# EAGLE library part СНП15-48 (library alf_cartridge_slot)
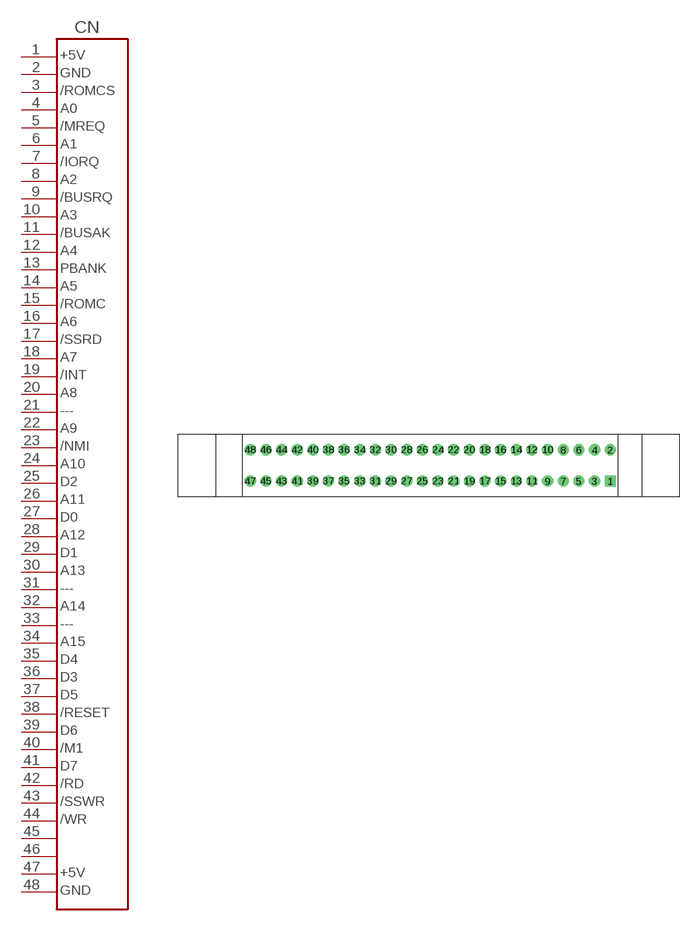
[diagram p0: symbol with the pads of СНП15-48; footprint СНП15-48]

Designator prefix CN

## СНП15-48  [СНП15-48]
1  1
2  2
3  3
4  4
5  5
6  6
7  7
8  8
9  9
10  10
11  11
12  12
13  13
14  14
15  15
16  16
17  17
18  18
19  19
20  20
21  21
22  22
23  23
24  24
25  25
26  26
27  27
28  28
29  29
30  30
31  31
32  32
33  33
34  34
35  35
36  36
37  37
38  38
39  39
40  40
41  41
42  42
43  43
44  44
45  45
46  46
47  47
48  48

## Footprint СНП15-48 (pad centres in mm)
drill 1 pad 1.778 square: 1 29,-2.5
drill 1 pad 1.778: 2 29,2.5; 3 26.5,-2.5; 4 26.5,2.5; 5 24,-2.5; 6 24,2.5; 7 21.5,-2.5; 8 21.5,2.5; 9 19,-2.5; 10 19,2.5; 11 16.5,-2.5; 12 16.5,2.5; 13 14,-2.5; 14 14,2.5; 15 11.5,-2.5; 16 11.5,2.5; 17 9,-2.5; 18 9,2.5; 19 6.5,-2.5; 20 6.5,2.5; 21 4,-2.5; 22 4,2.5; 23 1.5,-2.5; 24 1.5,2.5; 25 -1,-2.5; 26 -1,2.5; 27 -3.5,-2.5; 28 -3.5,2.5; 29 -6,-2.5; 30 -6,2.5; 31 -8.5,-2.5; 32 -8.5,2.5; 33 -11,-2.5; 34 -11,2.5; 35 -13.5,-2.5; 36 -13.5,2.5; 37 -16,-2.5; 38 -16,2.5; 39 -18.5,-2.5; 40 -18.5,2.5; 41 -21,-2.5; 42 -21,2.5; 43 -23.5,-2.5; 44 -23.5,2.5; 45 -26,-2.5; 46 -26,2.5; 47 -28.5,-2.5; 48 -28.5,2.5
